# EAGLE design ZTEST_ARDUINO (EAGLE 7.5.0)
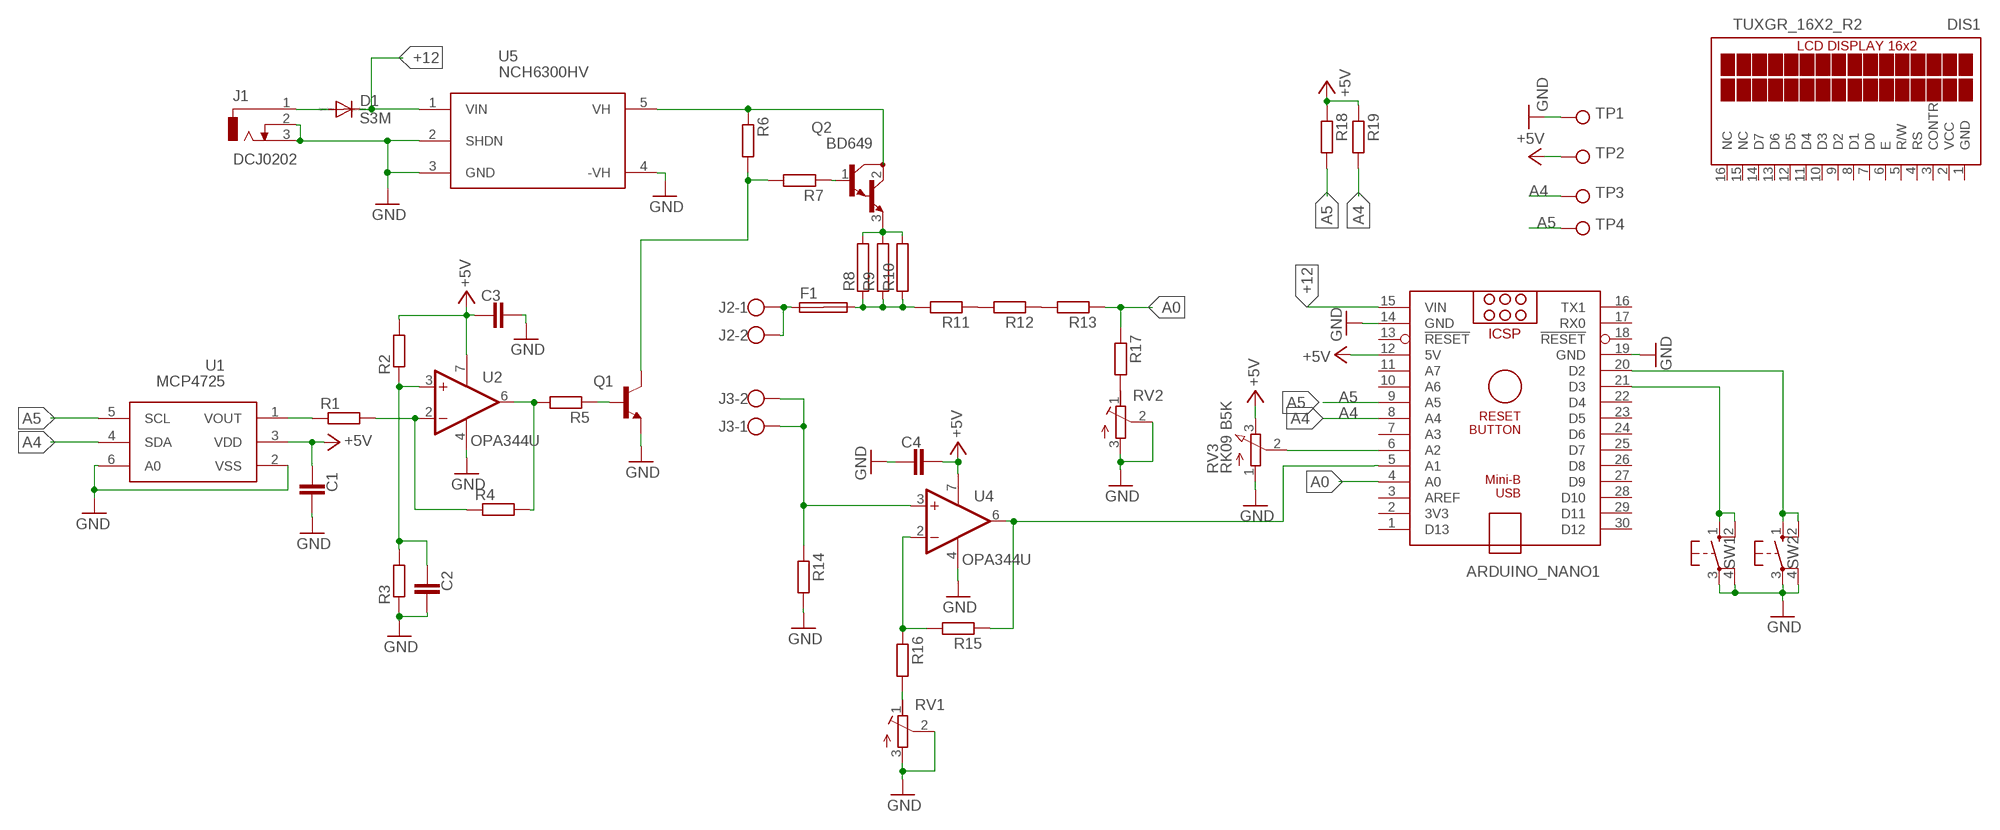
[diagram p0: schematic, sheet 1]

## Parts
ARDUINO_NANO1  ARDUINO_NANO  [ARDUINO_NANO]
C1  C-EUC1206  [C1206]
C2  C-EUC1206  [C1206]
C3  C-EUC1206  [C1206]
C4  C-EUC1206  [C1206]
D1  S3M  [SMC]
DIS1  TUXGR_16X2_R2  [TUXGR_16X2_R2]
F1  SHK20L  [SHK20L]
J1  DCJ0202  [DCJ0202]
J2  W237-102  [W237-102]
J3  W237-102  [W237-102]
Q1  -NPN-TO92-EBC  [TO92-EBC]
Q2  BD649  [TO220]
R1  R-EU_R1206  [R1206]
R2  R-EU_R1206  [R1206]
R3  R-EU_R1206  [R1206]
R4  R-EU_R1206  [R1206]
R5  R-EU_R1206  [R1206]
R6  R-EU_R1206  [R1206]
R7  R-EU_R1206  [R1206]
R8  RAC05  [AC05]
R9  RAC05  [AC05]
R10  RAC05  [AC05]
R11  R-EU_R1206  [R1206]
R12  R-EU_R1206  [R1206]
R13  R-EU_R1206  [R1206]
R14  R-EU_R1206  [R1206]
R15  R-EU_R1206  [R1206]
R16  R-EU_R1206  [R1206]
R17  R-EU_R1206  [R1206]
R18  R-EU_R1206  [R1206]
R19  R-EU_R1206  [R1206]
RV1  R-TRIMM-3386-F  [R-TRIMM-3386F]
RV2  R-TRIMM-3386-F  [R-TRIMM-3386F]
RV3  RK09 B5K  PV09A  [PTV09]
SW1  40-XX  [B3F-40XX]
SW2  40-XX  [B3F-40XX]
TP1  TPPAD1-13Y  [P1-13Y]
TP2  TPPAD1-13Y  [P1-13Y]
TP3  TPPAD1-13Y  [P1-13Y]
TP4  TPPAD1-13Y  [P1-13Y]
U1  MCP4725  [SOT23-6]
U2  OPA344U  [SO08]
U4  OPA344U  [SO08]
U5  NCH6300HV  [NCH6300]

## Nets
+5V: ARDUINO_NANO1.12(5V) C1.1 C3.1 C4.2 R2.2 R18.1 R19.1 RV3.3(E) TP2.TP U1.3(VDD) U2.7(V+) U4.7(V+)
+12: ARDUINO_NANO1.15(VIN) D1.C U5.1(VIN)
A0: ARDUINO_NANO1.4(A0) R13.1 R17.1
A4: ARDUINO_NANO1.8(A4) R19.2 TP3.TP U1.4(SDA)
A5: ARDUINO_NANO1.9(A5) R18.2 TP4.TP U1.5(SCL)
GND: ARDUINO_NANO1.14(GND) ARDUINO_NANO1.19(GND) C1.2 C2.2 C3.2 C4.1 J1.2 J1.3 Q1.E R3.1 R14.2 RV1.2(S) RV1.3(E) RV2.2(S) RV2.3(E) RV3.1(A) SW1.3(P) SW1.4(P1) SW2.3(P) SW2.4(P1) TP1.TP U1.2(VSS) U1.6(A0) U2.4(V-) U4.4(V-) U5.2(SHDN) U5.3(GND) U5.4(-VH)
N$1: Q2.2(C) R6.1 U5.5(VH)
N$2: D1.A J1.1
N$3: R1.1 U1.1(VOUT)
N$4: R1.2 R4.1 U2.2(-IN)
N$5: C2.1 R2.1 R3.2 U2.3(+IN)
N$6: Q2.3(E) R8.2 R9.2 R10.2
N$7: F1.2A R8.1 R9.1 R10.1 R11.2
N$8: Q1.C R6.2 R7.2
N$9: R17.2 RV2.1(A)
N$10: Q1.B R5.1
N$11: Q2.1(B) R7.1
N$12: F1.1A J2.1 J2.2
N$13: R4.2 R5.2 U2.6(OUT)
N$14: R11.1 R12.2
N$15: R12.1 R13.2
N$16: ARDUINO_NANO1.6(A2) RV3.2(S)
N$17: J3.1 J3.2 R14.1 U4.3(+IN)
N$18: R15.2 R16.1 U4.2(-IN)
N$19: ARDUINO_NANO1.5(A1) R15.1 U4.6(OUT)
N$20: R16.2 RV1.1(A)
N$21: ARDUINO_NANO1.21(D3) SW1.1(S) SW1.2(S1)
N$22: ARDUINO_NANO1.20(D2) SW2.1(S) SW2.2(S1)
Unconnected: ARDUINO_NANO1.1(D13) ARDUINO_NANO1.2(3V3) ARDUINO_NANO1.3(AREF) ARDUINO_NANO1.7(A3) ARDUINO_NANO1.10(A6) ARDUINO_NANO1.11(A7) ARDUINO_NANO1.13(!RESET) ARDUINO_NANO1.16(TX1) ARDUINO_NANO1.17(RX0) ARDUINO_NANO1.18(!RESET) ARDUINO_NANO1.22(D4) ARDUINO_NANO1.23(D5) ARDUINO_NANO1.24(D6) ARDUINO_NANO1.25(D7) ARDUINO_NANO1.26(D8) ARDUINO_NANO1.27(D9) ARDUINO_NANO1.28(D10) ARDUINO_NANO1.29(D11) ARDUINO_NANO1.30(D12) DIS1.3(CONTR) DIS1.4(RS) DIS1.5(R/W) DIS1.6(E) DIS1.7(D0) DIS1.8(D1) DIS1.9(D2) DIS1.10(D3) DIS1.11(D4) DIS1.12(D5) DIS1.13(D6) DIS1.14(D7) DIS1.15(NC) DIS1.16(NC) F1.1B F1.2B

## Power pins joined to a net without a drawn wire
GND: DIS1.1(GND)
VCC: DIS1.2(VCC)

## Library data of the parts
ARDUINO_NANO1 = ArduinoNanoV30:ARDUINO_NANO: Arduino Nano V3.0 Overview: The Arduino Nano is a small, complete, and breadboard-friendly board based on the ATmega328 (Arduino Nano 3.x) or ATmega168 (Arduino Nano 2.x). It has more or less the same functionality of the Arduino Duemilanove, but in a different package. It lacks only a DC power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
C1-C4 = rcl:C-EU: CAPACITOR, European symbol
D1 = diode:S3M
DIS1 = display-lcd:TUXGR_16X2_R2: Tuxgraphics LCD display 16x2 characters reflective, without background light Source: tuxgr_12x2_r2.pdf; OC_FARNELL: unknown; OC_NEWARK: unknown
F1 = fuse:SHK20L: FUSE HOLDER 5 x 20 mm, SH contact, SHH1 Schukat, E1073 Buerklin; OC_FARNELL: unknown; OC_NEWARK: unknown
J1 = con-jack:DCJ0202: DC POWER JACK Source: DCJ0202.pdf; OC_FARNELL: unknown; OC_NEWARK: unknown
J2 J3 = con-wago-500:W237-102: WAGO SCREW CLAMP; MPN: 237-102; OC_FARNELL: unknown; OC_NEWARK: 70K9898
Q1 = transistor-neu-to92:*-NPN-: NPN Transistror
Q2 = transistor:BD649: NPN BIPOLAR DARLINGTON TRANSISTOR
R1-R7 R11-R19 = rcl:R-EU_: RESISTOR, European symbol
R8-R10 = resistor-power:R: Power Resitor; OC_FARNELL: unknown; OC_NEWARK: unknown
RV1 RV2 = rcl:R-TRIMM-3386-F
RV3 = pot:PV09A
SW1 SW2 = switch-omron:40-XX: OMRON SWITCH; MF: OMRON COMPONENTS USA; MPN: B3F-4000; OC_FARNELL: 176434; OC_NEWARK: 36K3105
TP1-TP4 = testpad:TP: Test pad
U1 = linear:MCP4725
U2 U4 = linear:OPA*: Single Operational Amplifier Low Power, Single-Supply, Rail-To-Rail Operational Amplifier Source: http://focus.ti.com/lit/ds/symlink/opa2345.pdf
U5 = dc-dc-converter:NCH6300HV

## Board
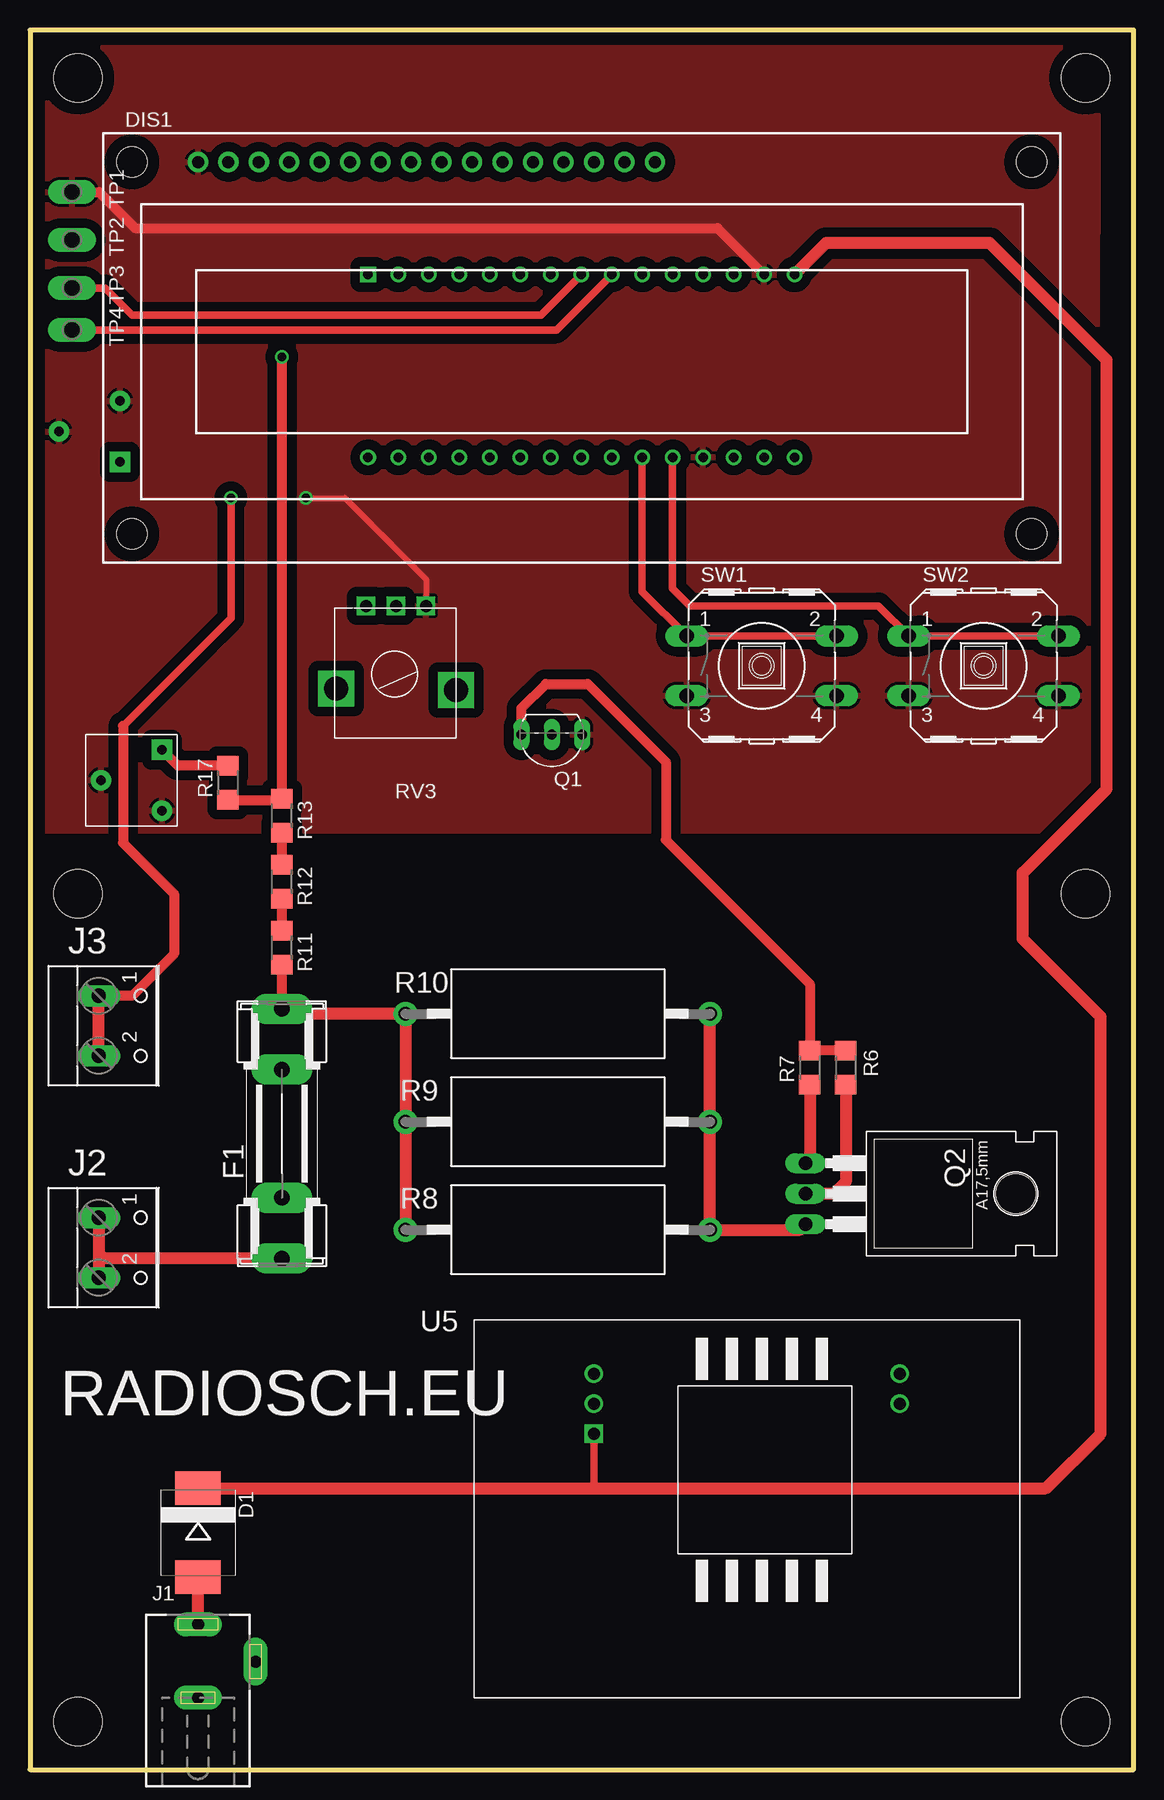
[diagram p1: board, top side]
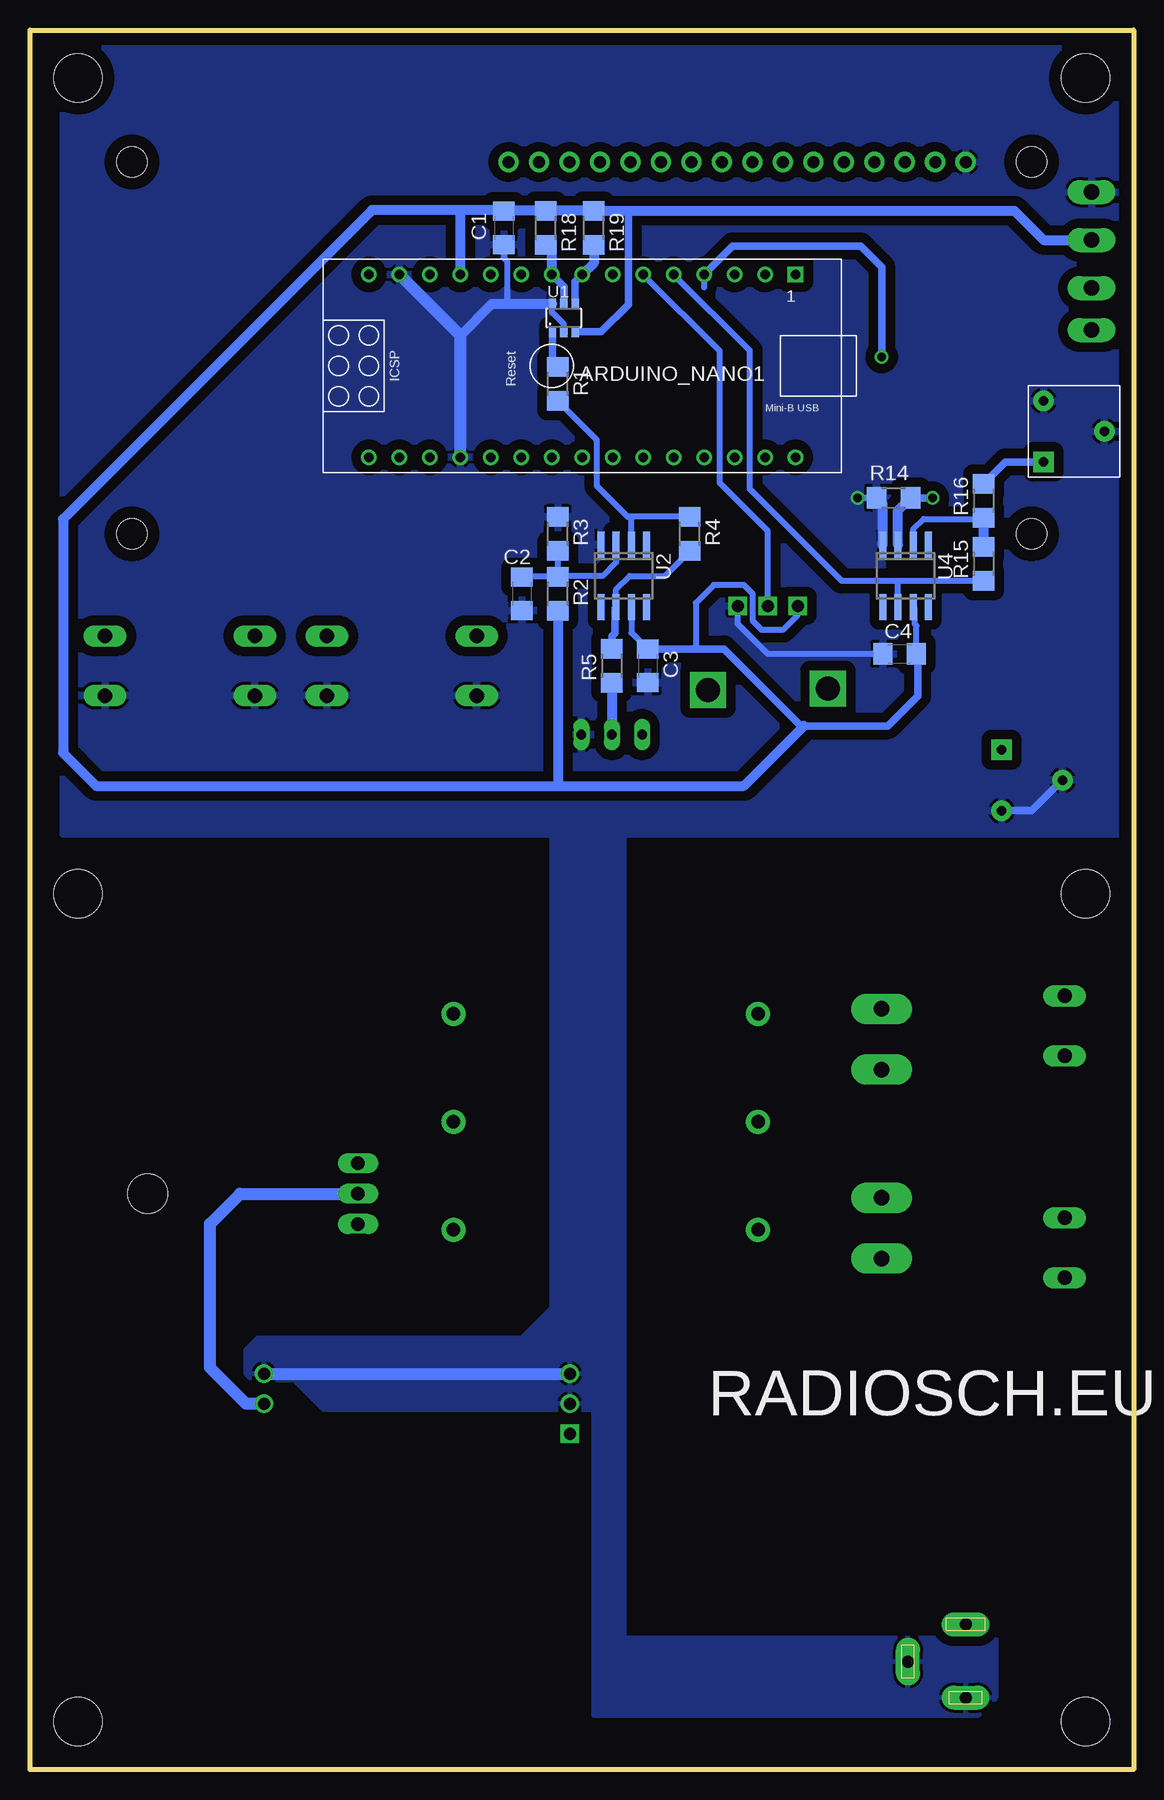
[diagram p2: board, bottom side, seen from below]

Size 92 x 145 mm. Coordinates in mm from the lower left corner, seen from the top.
Outline: 0,0 92,0 92,145 0,145 0,0
Copper layers (1*16): Top 0.035mm / dielectric 1.5mm / Bottom 0.035mm
Design rules "default": minimum track width 10mil, minimum drill 24mil, track to track 8mil, track to pad 8mil, pad to pad 8mil, via to via 8mil, smd to smd 8mil, copper to edge 40mil, drill to drill 8mil, minimum pad ring 10mil, minimum via ring 8mil, stop-mask expansion 4mil, vias tented up to drill 0mil, thermal gap 10mil
Holes 4 mm at 88,4 4,4 4,141 88,141 4,73 88,73

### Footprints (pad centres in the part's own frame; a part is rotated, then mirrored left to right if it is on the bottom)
ARDUINO_NANO = drill 0.8 square: 1 -20.32,-7.62 | drill 0.8: 2 -17.78,-7.62; 3 -15.24,-7.62; 4 -12.7,-7.62; 5 -10.16,-7.62; 6 -7.62,-7.62; 7 -5.08,-7.62; 8 -2.54,-7.62; 9 0,-7.62; 10 2.54,-7.62; 11 5.08,-7.62; 12 7.62,-7.62; 13 10.16,-7.62; 14 12.7,-7.62; 15 15.24,-7.62; 16 15.24,7.62; 17 12.7,7.62; 18 10.16,7.62; 19 7.62,7.62; 20 5.08,7.62; 21 2.54,7.62; 22 0,7.62; 23 -2.54,7.62; 24 -5.08,7.62; 25 -7.62,7.62; 26 -10.16,7.62; 27 -12.7,7.62; 28 -15.24,7.62; 29 -17.78,7.62; 30 -20.32,7.62
C1206 = smd 1.6 x 1.8: 1 -1.4,0; 2 1.4,0
SMC = smd 2.8 x 3.8: A 3.7,0; C -3.7,0
TUXGR_16X2_R2 = drill 1 pad 1.676: 1 -32,15.5; 2 -29.46,15.5; 3 -26.92,15.5; 4 -24.38,15.5; 5 -21.84,15.5; 6 -19.3,15.5; 7 -16.76,15.5; 8 -14.22,15.5; 9 -11.68,15.5; 10 -9.14,15.5; 11 -6.6,15.5; 12 -4.06,15.5; 13 -1.52,15.5; 14 1.02,15.5; 15 3.56,15.5; 16 6.1,15.5 | hole 2.5: -37.5,-15.5; 37.5,-15.5; -37.5,15.5; 37.5,15.5
SHK20L = drill 1.321 pad 2.54 long: 1A -10.414,0; 1B -5.334,0; 2A 10.414,0; 2B 5.334,0
DCJ0202 = drill 1 pad 2 long: 1 0,3.1; 2 4.8,0; 3 0,-3
W237-102 = drill 1.194 long: 1 -2.5,-1.27; 2 2.5,-1.27
TO92-EBC = drill 0.813 long: B 0,-1.27; C 2.54,-1.27; E -2.54,-1.27
TO220 = drill 1.118 long: 1 -2.54,-6.35; 2 0,-6.35; 3 2.54,-6.35 | hole 3.302: 0,11.176
R1206 = smd 1.6 x 1.803: 1 -1.422,0; 2 1.422,0
AC05 = drill 1.1 pad 2: 1 -12.7,0; 2 12.7,0
R-TRIMM-3386F = drill 0.8 pad 1.676 square: 1 0,0 | drill 0.8 pad 1.676: 2 5.08,2.54; 3 0,5.08
PTV09 = drill 1 square: 1 -2.5,0; 2 0,0; 3 2.5,0 | drill 2 square: P$4 -5,7; P$5 5,6.9
B3F-40XX = drill 1.194 long: 1 -6.248,2.489; 2 6.248,2.489; 3 -6.248,-2.489; 4 6.248,-2.489
P1-13Y = drill 1.321 pad 1.905 long: TP 0,0
SOT23-6 = smd 0.6 x 0.9: 1 -0.95,-1.15; 2 0,-1.15; 3 0.95,-1.15; 4 0.95,1.15; 5 0,1.15; 6 -0.95,1.15
SO08 = smd 0.6 x 2.2: 1 -1.905,-2.6; 2 -0.635,-2.6; 3 0.635,-2.6; 4 1.905,-2.6; 5 1.905,2.6; 6 0.635,2.6; 7 -0.635,2.6; 8 -1.905,2.6
NCH6300 = drill 1 square: 1 10,22 | drill 1: 2 10,24.5; 3 10,27; 4 35.5,27; 5 35.5,24.5

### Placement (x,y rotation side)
ARDUINO_NANO1  48.5,117 180 bottom
C1  52.5,128.5 270 bottom
C2  51,98 270 bottom
C3  40.5,92 270 bottom
C4  19.5,93 0 bottom
D1  14,19.75 270 top
DIS1  46,118.5 0 top
F1  21,53 90 top
J1  14,9 0 top
J2  7,43.5 270 top
J3  7,62 270 top
Q1  43.5,85 180 top
Q2  71,48 270 top
R1  48,115.5 270 bottom
R2  48,98 270 bottom
R3  48,103 270 bottom
R4  37,103 270 bottom
R5  43.5,92 90 bottom
R6  68,58.5 90 top
R7  65,58.5 90 top
R8  44,45 0 top
R9  44,54 0 top
R10  44,63 0 top
R11  21,68.5 270 top
R12  21,74 270 top
R13  21,79.5 270 top
R14  20,106 180 bottom
R15  12.5,100.5 90 bottom
R16  12.5,105.75 90 bottom
R17  16.5,82.25 90 top
R18  49,128.5 270 bottom
R19  45,128.5 270 bottom
RV1  7.5,109 0 bottom
RV2  11,85 180 top
RV3  30.5,97 180 top
SW1  61,92 0 top
SW2  79.5,92 0 top
TP1  3.5,131.5 90 top
TP2  3.5,127.5 90 top
TP3  3.5,123.5 90 top
TP4  3.5,120 90 top
U1  47.5,121 0 bottom
U2  42.5,99.5 180 bottom
U4  19,99.5 180 bottom
U5  37,6 0 top

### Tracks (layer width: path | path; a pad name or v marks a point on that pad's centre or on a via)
+5V
  Bottom 0.5: C4.2 18.1,95.35 18.25,95.5 18.25,96.78 U4.7 | U2.7 41.86,94.77 C3.1 | RV3.3 28,96.25 29.25,95 31,95 31.75,95.75 31.75,98 32.5,98.75 35,98.75 36.5,97.25 36.5,93.65 36.25,93.4
  Bottom 0.61: C3.1 36.25,93.4 34.15,93.4 27.75,87 27.5,87 20.5,87 18,89.5 18,92.9 C4.2 | U1.3 44.4,119.85 42.12,122.12 42.12,129.8 42.25,129.92
  Bottom 0.813: ARDUINO_NANO1.12 56.12,129.88 56,130 | TP2.TP 7.5,127.5 9.92,129.92 42.25,129.92 R19.1 R18.1 52.48,129.92 C1.1 52.6,130 56,130 | 56,130 63.5,130 89.25,104.25 89.25,84.75 86.5,82 48.25,82 | 48.25,82 32.5,82 27.5,87 | R2.2 48,82.25 48.25,82
+12
  Top 0.61: U5.1 47,23.45
  Top 1.016: D1.C 47,23.45 84.7,23.45 89.25,28 89.25,62.75 82.75,69.25 82.75,74.75 89.75,81.75 89.75,117.5 80,127.25 66.37,127.25 ARDUINO_NANO1.15
A0  (via drill 0.7)
  Top 0.813: R17.1 20.91,80.83 R13.1 v21,117.75
  Bottom 0.5: ARDUINO_NANO1.4 35.8,123.55
  Bottom 0.61: v21,117.75 21,125.25 22.75,127 33.42,127 ARDUINO_NANO1.4
A4
  Top 0.61: TP3.TP 6.25,123.5 8.5,121.25 42.59,121.25 ARDUINO_NANO1.8
  Bottom 0.61: U1.4 46.55,124.03 ARDUINO_NANO1.8
  Bottom 0.813: R19.2 45,125.58 ARDUINO_NANO1.8
A5
  Top 0.61: TP4.TP 43.88,120 ARDUINO_NANO1.9
  Bottom 0.61: U1.5 47.5,123.62 ARDUINO_NANO1.9
  Bottom 0.813: ARDUINO_NANO1.9 48.5,126.58 R18.2
GND  (via drill 0.7)
  Top 0.5: v23,106 26.25,106 33,99.25 RV3.1
  Top 0.813: TP1.TP 5.75,131.5 8.75,128.5 57.32,128.5 ARDUINO_NANO1.14
  Bottom 0.5: C1.2 52.5,126 52.25,125.75 52.25,122.15 | U1.2 47.5,120.5 48.5,121.5 48.5,122.1 U1.6 | C4.1 30.5,93 33,95.5 RV3.1 | U4.4 20.91,105.41 21.5,106 v23,106
  Bottom 0.61: RV2.3 8.46,79.92 RV2.2
  Bottom 0.813: U1.6 52.25,122.15 53.51,122.15 56.12,119.54 | U4.4 20.91,105.48 R14.2
  Bottom 1.016: ARDUINO_NANO1.19 56.12,119.54 ARDUINO_NANO1.14 | U5.4 U5.3
  pour Top (isolate 0.813): 1,144.5 89,144.5 88.75,78.25 0.75,78.25
  pour Bottom (isolate 0.813): 1.25,144 89.25,144 89.25,78 1.25,78
  pour Bottom (isolate 0.813): 13,4.5 45,4.5 45,30 67.5,30 70,32.5 73.5,32.5 74,33 74,35 73,36 51,36 48.5,38.5 48.5,79.5 42.5,79.5 42.5,11 11.5,11 11.5,6
N$1
  Top 1.016: R6.1 68,49 67,48 Q2.2
  Bottom 1.016: U5.5 74,30.5 77,33.5 77,45.5 74.5,48 Q2.2
N$2
  Top 1.016: J1.1 D1.A
N$3
  Bottom 0.61: U1.1 48.45,117.37 R1.1
N$4
  Bottom 0.5: R4.1 41.75,104.42 | 41.75,104.42 42.17,104.42 44.75,107 44.75,110.83 R1.2 | U2.2 41.86,104.31 41.75,104.42
N$5
  Bottom 0.5: R2.1 R3.2 | U2.3 43.14,100.61 44.25,99.5 47.92,99.5 R2.1 | R2.1 50.98,99.42 C2.1
N$6
  Top 1.016: R10.2 R9.2 R8.2 64.19,45 Q2.3
N$7
  Top 0.813: F1.2A R11.2
  Top 1.016: F1.2A 21.41,63 R10.1 R9.1 R8.1
N$8
  Top 0.813: Q1.C 40.96,88.46 43,90.5 46.5,90.5 53,84 53,77.5 65,65.5 R7.2 R6.2
N$9
  Top 0.813: R17.2 12.33,83.67 RV2.1
N$10
  Bottom 0.813: R5.1 Q1.B
N$11
  Top 1.016: R7.1 65,50.89 Q2.1
N$12
  Top 1.016: J2.1 5.73,43 | 5.73,43 J2.2 | F1.1A 6.14,42.59 5.73,43
N$13
  Bottom 0.5: U2.6 43.14,98.36 42,99.5 39.08,99.5 R4.2
  Bottom 0.61: R5.2 43.5,94.5 43.25,94.75 43.25,96.78 U2.6
N$14
  Top 0.813: R11.1 R12.2
N$15
  Top 0.813: R12.1 R13.2
N$16
  Bottom 0.5: RV3.2 30.5,103.25 34.5,107.25 34.5,118.24 ARDUINO_NANO1.6
N$17  (via drill 0.7)
  Top 0.61: 7.75,87 16.75,96 v16.75,106
  Top 0.813: 7.75,87 7.75,77.25 12,73 12,68 8.5,64.5 J3.1
  Top 1.016: J3.2 J3.1
  Bottom 0.61: v16.75,106 R14.1
  Bottom 0.813: U4.3 19.63,104.94 R14.1
N$18
  Bottom 0.5: U4.2 18.37,103.39 17.5,104.25 12.58,104.25 R16.1
  Bottom 0.813: R15.2 R16.1
N$19
  Bottom 0.5: R15.1 19.5,99.08 | 19.5,99.08 24.33,99.08 32,106.75 32,118.28 ARDUINO_NANO1.5 | U4.6 19.63,98.94 19.5,99.08
N$20
  Bottom 0.61: RV1.1 10.67,109 R16.2
N$21
  Top 0.61: SW1.2 SW1.1 51.04,98.2 ARDUINO_NANO1.21
N$22
  Top 0.61: ARDUINO_NANO1.20 53.58,98.42 55,97 70.74,97 SW2.1 SW2.2

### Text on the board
tPlace: RADIOSCH.EU
bPlace: RADIOSCH.EU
